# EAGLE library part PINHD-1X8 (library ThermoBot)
PIN HEADER
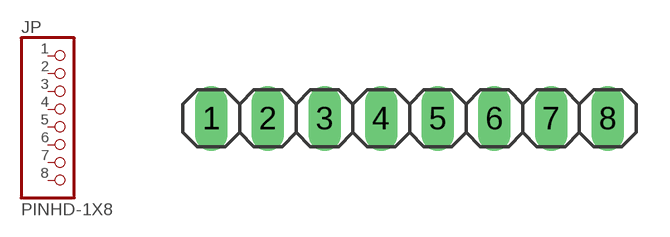
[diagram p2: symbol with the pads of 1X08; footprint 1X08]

Designator prefix JP

## PINHD-1X8TH  [1X08]
1  1  pas
2  2  pas
3  3  pas
4  4  pas
5  5  pas
6  6  pas
7  7  pas
8  8  pas

## Footprint 1X08 (pad centres in mm)
drill 0.95 pad 1.422 long: 1 -8.89,0; 2 -6.35,0; 3 -3.81,0; 4 -1.27,0; 5 1.27,0; 6 3.81,0; 7 6.35,0; 8 8.89,0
